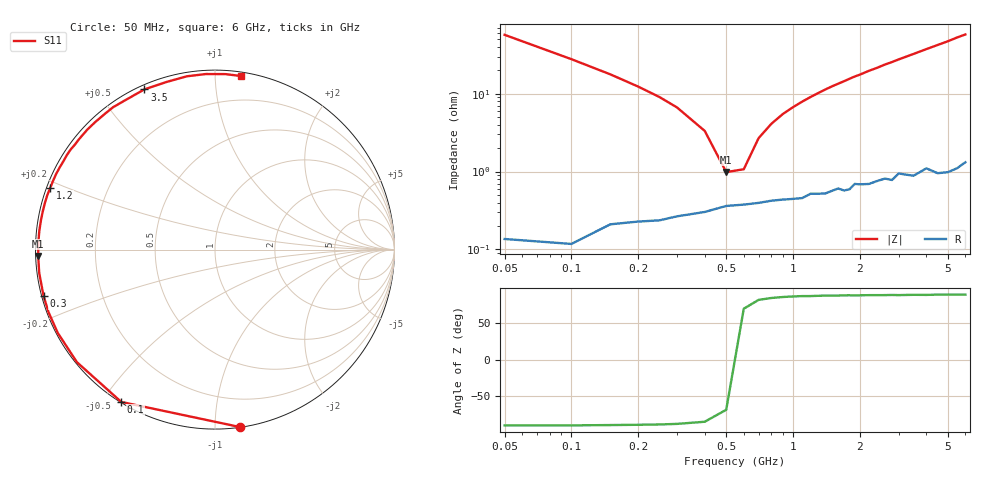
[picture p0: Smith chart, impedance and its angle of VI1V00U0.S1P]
! Infineon Technologies  Discrete & RF Semiconductors
! BB 804
! Si Tuning Diode in SOT23
! VR = 1 V
! S-Parameters:  July  1999
# GHz  S  MA  R  50
!  f  S11
! GHz  MAG  ANG
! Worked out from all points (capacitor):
!   34 points, 50 MHz to 6 GHz, reference 50 ohm
!   read as one part to ground: C = 55.1 pF near 50 MHz
!   lowest |Z| = 985 mohm at 500 MHz (marker M1)
!   series resonance near 547.7 MHz, so ESL is about 1.5 nH
!   S11 on the Smith chart (normalised r, x): 50 MHz: 0.00, -1.15; 100 MHz: 0.00, -0.56; 300 MHz: 0.01, -0.13; 1.2 GHz: 0.01, +0.18; 3.5 GHz: 0.02, +0.65; 6 GHz: 0.03, +1.16
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0.05  0.9977 -82.1
0.1  0.9964 -121.6
0.15  0.9926 -140.8
0.2  0.9915 -152.1
0.25  0.9909 -159.4
0.3  0.9896 -164.8
0.4  0.988 -172.4
0.5  0.9857 -177.9
0.6  0.9851 177.7
0.7  0.9843 173.9
0.8  0.9834 170.6
1  0.9827 164.7
1.2  0.9801 159.4
1.4  0.9803 154.4
1.6  0.9777 149.8
1.7  0.9791 147.6
1.9  0.9753 143.1
2.2  0.9763 136.9
2.4  0.9748 133.2
2.6  0.9738 129.1
2.8  0.9756 125.7
3  0.9715 122.0
3.5  0.9755 113.8
4  0.9723 106.1
4.5  0.9781 99.2
5  0.9795 93.0
5.5  0.9795 86.6
6  0.9778 81.5
